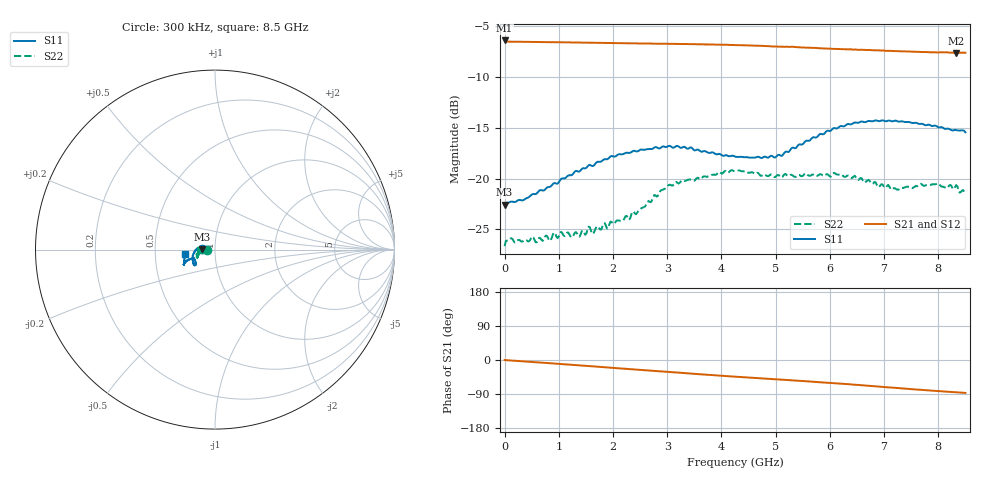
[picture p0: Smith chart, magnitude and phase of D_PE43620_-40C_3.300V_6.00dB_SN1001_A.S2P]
! device id: pe43620
! dir: c:\dsa\pe43620\data\pe43620\-40c\3p300v\06p00db
! Serial: 1001
! Insertion: A
! Temp: -40C
! VDD: 3.300V
! Attenuation Step: 6.00dB
! IDD: 7.429218e-03mA
! FILE NAME
! DATE 10-22-2008 14:40:15
! CORRECTED  DATA
#  Hz  S  RI  R  50.00
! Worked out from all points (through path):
!   401 points, 300 kHz to 8.5 GHz, reference 50 ohm
!   highest |S21| = -6.40 dB at 300 kHz (marker M1); lowest = -7.6 dB at 8.33 GHz (marker M2)
!   group delay of S21, straight-line fit = 28.2 ps
!   lowest |S11| = -22.6 dB at 300 kHz (marker M3), VSWR 1.16, Z = 43.1 + j0.059 ohm
!   |S11| at or under -10 dB: start of sweep to end of sweep
!   |S22| runs from -26.7 to -19.2 dB; largest |S21 - S12| = 0.0022
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300000  -0.0743 0.000681  0.4784 -0.000646  0.477 0.000972  -0.0465 -0.000187
1.065463e8  -0.0768 0.00145  0.4715 -0.01  0.472 -0.00988  -0.0507 -0.00144
3.615373e8  -0.0784 0.00747  0.4701 -0.0306  0.4704 -0.0307  -0.0497 -0.00139
1.424e9  -0.1112 -0.00654  0.4519 -0.1183  0.4522 -0.1183  -0.0544 -0.0091
1.551495e9  -0.1156 -0.0133  0.4486 -0.1284  0.4488 -0.1285  -0.0568 -0.0116
1.636492e9  -0.1143 -0.0162  0.4459 -0.1352  0.4465 -0.1353  -0.0525 -0.0107
1.97648e9  -0.1241 -0.0362  0.4356 -0.1625  0.436 -0.1623  -0.0595 -0.0143
2.295219e9  -0.1233 -0.0517  0.4238 -0.188  0.424 -0.1877  -0.0612 -0.0136
2.8477e9  -0.1182 -0.0761  0.4006 -0.2285  0.401 -0.2281  -0.0827 -0.0159
3.017694e9  -0.1186 -0.0824  0.3928 -0.2408  0.393 -0.2408  -0.0898 -0.0225
3.293934e9  -0.1142 -0.0861  0.3796 -0.2589  0.3796 -0.2591  -0.0931 -0.0303
4.25015e9  -0.1083 -0.0693  0.3266 -0.3153  0.3269 -0.3156  -0.1008 -0.0418
4.993874e9  -0.1178 -0.0476  0.2821 -0.3463  0.2809 -0.3468  -0.0956 -0.0349
5.67385e9  -0.1483 -0.0563  0.2378 -0.3695  0.2384 -0.3704  -0.1009 -0.0278
6.098835e9  -0.1633 -0.0686  0.2073 -0.3821  0.2088 -0.3813  -0.1017 -0.0301
6.460072e9  -0.1723 -0.0776  0.1811 -0.3918  0.1819 -0.3919  -0.0996 -0.0273
7.09755e9  -0.1742 -0.0833  0.1295 -0.4057  0.1288 -0.4056  -0.0895 -0.0182
7.246294e9  -0.1731 -0.082  0.1173 -0.4072  0.117 -0.4078  -0.0874 -0.0121
7.968769e9  -0.1716 -0.058  0.0604 -0.4135  0.0594 -0.4134  -0.0939 -0.00794
8.117514e9  -0.1692 -0.0476  0.0495 -0.4149  0.0495 -0.4139  -0.0903 -0.00724
8.330006e9  -0.17 -0.0345  0.0348 -0.414  0.0341 -0.4145  -0.0925 -0.00762
8.5e9  -0.167 -0.0258  0.023 -0.4158  0.0227 -0.4166  -0.0851 -0.00389
